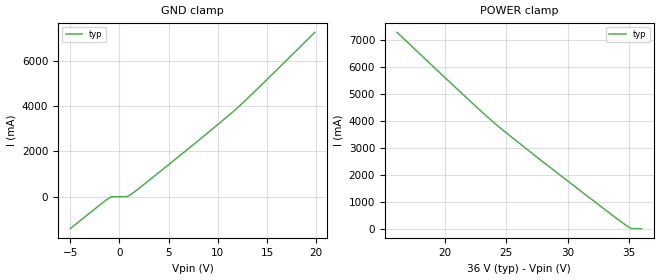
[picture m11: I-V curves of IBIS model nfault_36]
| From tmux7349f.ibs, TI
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| nfault_36
[Model]   nfault_36
Model_type   Input
Vinl = 0.8
Vinh = 1.3
|   typ   min   max
C_comp   NA   NA
[Voltage Range]   36   NA   NA
[Temperature Range]   27   NA   NA
[Power Clamp Reference]   36   NA   NA
[GND Clamp Reference]   0   NA   NA
[GND Clamp]
|   Voltage   I(typ)   I(min)   I(max)
-5V       -1.413A    NA         NA
-1.687V   -263.7mA   NA         NA
-858.6mV  -8.928mA   NA         NA
798mV     2.683mA    NA         NA
1.212V    105.9mA    NA         NA
3.697V    958.6mA    NA         NA
8.667V    2.705A     NA         NA
11.98V    3.916A     NA         NA
19.85V    7.255A     NA         NA
[POWER Clamp]
|   Voltage   I(typ)   I(min)   I(max)
16.12V    7.268A     NA         NA
22.75V    4.434A     NA         NA
24.82V    3.615A     NA         NA
28.13V    2.422A     NA         NA
34.76V    115.7mA    NA         NA
35.17V    5.14mA     NA         NA
36V       -7.684uA   NA         NA
